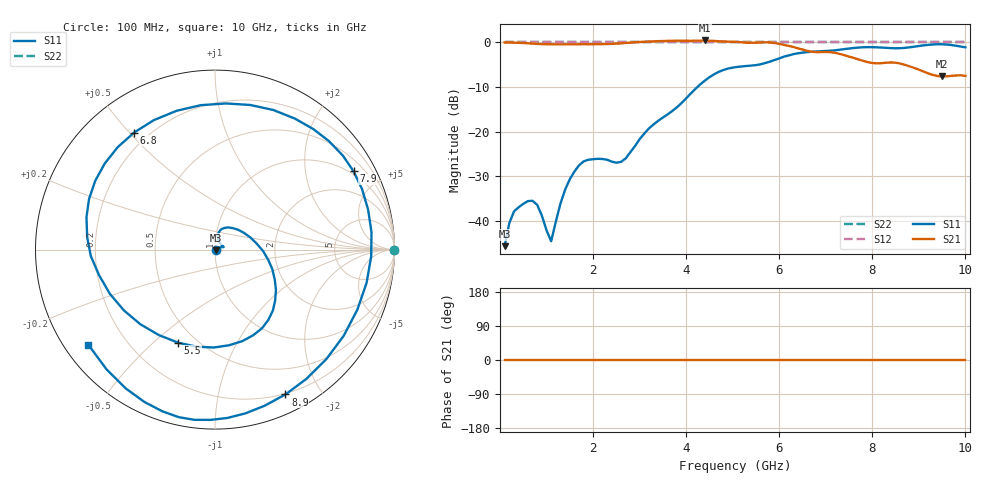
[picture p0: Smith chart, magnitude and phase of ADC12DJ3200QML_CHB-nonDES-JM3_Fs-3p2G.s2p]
!	Texas	"Instruments,"	Inc.
!	ADC12DJ3200	-	CH	B	S-Parameters	(DES	"Mode,"	Fs	=	3.2	"GSPS,"	25	degC	"case,"	15	degC	juntion)
!	Port	1	represents	the	100-ohm	differential	"input,"	Port	2	the	digital	output
!	freq	dbS11	angS11	dbS21	angS21	dbS12	angS12	dbS22	angS22
#	HZ	S	DB	R	100
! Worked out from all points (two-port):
!   100 points, 100 MHz to 10 GHz, reference 100 ohm
!   highest |S21| = 0.45 dB at 4.4 GHz (marker M1); lowest = -7.6 dB at 9.5 GHz (marker M2)
!   |S21| within 3 dB of the highest: start of sweep to 7.293 GHz
!   lowest |S11| = -45.7 dB at 100 MHz (marker M3), VSWR 1.01, Z = 101 - j0.758 ohm
!   |S11| at or under -10 dB: start of sweep to 4.241 GHz
!   |S22| runs from 0.0 to 0.0 dB; largest |S21 - S12| = 0.58
!   S11 on the Smith chart (normalised r, x): 100 MHz: 1.01, -0.01; 5.5 GHz: 0.40, -0.60; 6.8 GHz: 0.15, +0.52; 7.9 GHz: 0.88, +3.60; 8.9 GHz: 0.19, -1.58; 10 GHz: 0.07, -0.33
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1e8  -45.68 -46.3  0.00 0.0  0.00 0.0  0.00 0.0
3e8  -37.90 -64.5  -0.05 0.0  0.00 0.0  0.00 0.0
6e8  -35.57 -87.4  -0.18 0.0  0.00 0.0  0.00 0.0
8e8  -36.41 -87.8  -0.32 0.0  0.00 0.0  0.00 0.0
1.1e9  -44.57 -23.6  -0.40 0.0  0.00 0.0  0.00 0.0
1.4e9  -33.01 22.0  -0.41 0.0  0.00 0.0  0.00 0.0
1.8e9  -26.66 19.3  -0.39 0.0  0.00 0.0  0.00 0.0
2.6e9  -26.77 52.2  -0.21 0.0  0.00 0.0  0.00 0.0
3.4e9  -17.56 65.9  0.30 0.0  0.00 0.0  0.00 0.0
3.9e9  -13.60 18.7  0.38 0.0  0.00 0.0  0.00 0.0
4.4e9  -8.56 -26.8  0.45 0.0  0.00 0.0  0.00 0.0
5.1e9  -5.48 -73.4  0.13 0.0  0.00 0.0  0.00 0.0
5.5e9  -5.07 -111.6  -0.06 0.0  0.00 0.0  0.00 0.0
6.1e9  -3.19 -177.1  -0.54 0.0  0.00 0.0  0.00 0.0
6.7e9  -2.08 133.4  -2.09 0.0  0.00 0.0  0.00 0.0
6.8e9  -2.02 124.6  -2.16 0.0  0.00 0.0  0.00 0.0
7.3e9  -1.62 76.3  -2.56 0.0  0.00 0.0  0.00 0.0
7.9e9  -1.04 29.5  -4.40 0.0  0.00 0.0  0.00 0.0
8.4e9  -1.26 -12.4  -4.48 0.0  0.00 0.0  0.00 0.0
8.9e9  -0.94 -64.1  -5.70 0.0  0.00 0.0  0.00 0.0
9.5e9  -0.40 -102.2  -7.62 0.0  0.00 0.0  0.00 0.0
1e10  -1.08 -143.1  -7.49 0.0  0.00 0.0  0.00 0.0
